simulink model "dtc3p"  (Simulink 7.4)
settings: Solver=ode45  StartTime=0.0  StopTime=.03  MaxStep=2e-5  RelTol=1e-3
undefined symbols (not defined in the file or in its folder): a

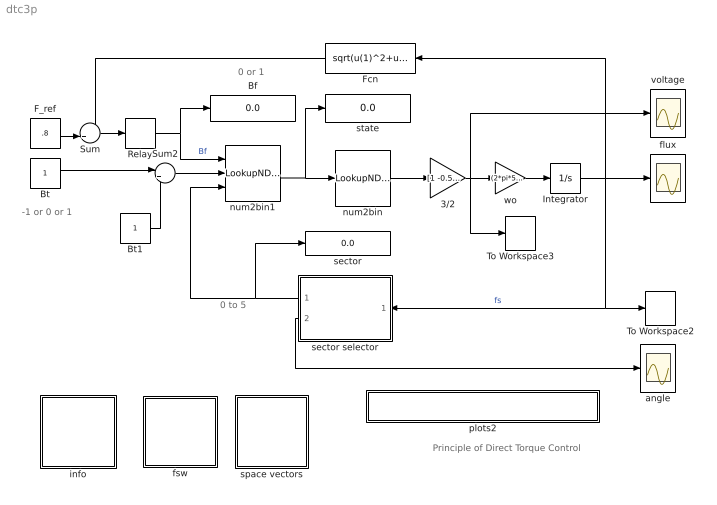
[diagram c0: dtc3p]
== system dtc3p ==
  note: Principle of Direct Torque Control
  note: -1 or 0 or 1
  note: 0 to 5
  note: 0 or 1
  3/2 : Gain  Gain=[1 -0.5 -0.5;0 sqrt(3)/2 -sqrt(3)/2]  Multiplication=Matrix(K*u)  ParameterDataType=sfix(16)  ParameterScaling=2^0  OutDataType=sfix(16)  OutScaling=2^0
  Bf : Display
  Bt : Constant  OutDataType=sfix(16)  OutScaling=2^0
  Bt1 : Constant  OutDataType=sfix(16)  OutScaling=2^0
  F_ref : Constant  Value=.8  OutDataType=sfix(16)  OutScaling=2^0
  Fcn : Fcn  Expr=sqrt(u(1)^2+u(2)^2)
  Integrator : Integrator  InitialCondition=[1 0]
  Relay : Relay  OnSwitchValue=.02  OffSwitchValue=-.02  OutDataType=sfix(16)  OutScaling=2^0
  Sum : Sum  Inputs=-+|  OutDataType=sfix(16)  OutScaling=2^0
  Sum2 : Sum  Inputs=|++  OutDataType=sfix(16)  OutScaling=2^0
  To Workspace2 : ToWorkspace  VariableName=f_ab  SampleTime=-1  SaveFormat=Array
  To Workspace3 : ToWorkspace  VariableName=f  SampleTime=-1  SaveFormat=Array
  angle : Scope
  flux : Scope
  fsw : Subsystem
  info : Subsystem
  num2bin : LookupNDDirect  InputsSelectThisObjectFromTable=Column  Table=[0 0 0;1 0 0;0 1 0;1 1 0;0 0 1;1 0 1;0 1 1;1 1 1]'  ActionForOutOfRangeInput=Error
  num2bin1 : LookupNDDirect  NumberOfTableDimensions=3  Table=a  ActionForOutOfRangeInput=Error
  plots2 : Subsystem
  sector : Display
  sector selector : Subsystem
  space vectors : Subsystem
  state : Display
  voltage : Scope
  wo : Gain  Gain=(2*pi*50)  ParameterDataType=sfix(16)  ParameterScaling=2^0  OutDataType=sfix(16)  OutScaling=2^0
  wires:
  num2bin1/1 -> state/1, num2bin/1
  num2bin/1 -> 3/2/1
  F_ref/1 -> Sum/2
  Sum/1 -> Relay/1
  Relay/1 -> Bf/1, num2bin1/1  "Bf"
  Fcn/1 -> Sum/1
  wo/1 -> Integrator/1
  3/2/1 -> wo/1, voltage/1, To Workspace3/1
  Integrator/1 -> Fcn/1, flux/1, sector selector/1(fs), To Workspace2/1  "fs"
  sector selector/1(sector) -> sector/1, num2bin1/3
  Sum2/1 -> num2bin1/2
  Bt/1 -> Sum2/1
  Bt1/1 -> Sum2/2
  sector selector/2(angle) -> angle/1

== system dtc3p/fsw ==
  note: Script files
  note: This collection of demonstrations is designed to illustrate the use of MATLAB for the simulation of the steady-state characteristics of ac machines under balanced and unbalanced conditions of operation.

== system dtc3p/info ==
  note: Principle of direct torque control of an induction motor
  note: This demo shows how to produce a rotating flux vector of specified magnitude F_ref using the principle of direct torque control: a) Bt = 1 establishes a positively rotating wave (counterclockwize) b) Bt = -1 establishes a negatively rotating wave (clockwize) c) Bt = 0 keeps the flux vector fixed in its original state Before running, double click the Switching Table block. Observe the effect of changing the magnitude of F_ref and/or wo (gain preceding the integrator) upon the speed (frequency) of the rotating space vector.

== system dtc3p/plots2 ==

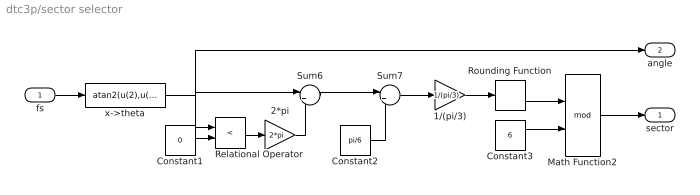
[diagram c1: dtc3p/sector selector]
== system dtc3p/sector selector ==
  fs : Inport  OutDataType=sfix(16)  OutScaling=2^0
  1/(pi/3) : Gain  Gain=1/(pi/3)  ParameterDataType=sfix(16)  ParameterScaling=2^0  OutDataType=sfix(16)  OutScaling=2^0
  2*pi : Gain  Gain=2*pi  ParameterDataType=sfix(16)  ParameterScaling=2^0  OutDataType=sfix(16)  OutScaling=2^0
  Constant1 : Constant  Value=0  OutDataType=sfix(16)  OutScaling=2^0
  Constant2 : Constant  Value=pi/6  OutDataType=sfix(16)  OutScaling=2^0
  Constant3 : Constant  Value=6  OutDataType=sfix(16)  OutScaling=2^0
  Math Function2 : Math  Operator=mod
  Relational Operator : RelationalOperator  Operator=<
  Rounding Function : Rounding
  Sum6 : Sum  Inputs=|++  OutDataType=sfix(16)  OutScaling=2^0
  Sum7 : Sum  Inputs=|++  OutDataType=sfix(16)  OutScaling=2^0
  x->theta : Fcn  Expr=atan2(u(2),u(1))
  sector : Outport
  angle : Outport  Port=2
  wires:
  Constant1/1 -> Relational Operator/2
  Relational Operator/1 -> 2*pi/1
  2*pi/1 -> Sum6/2
  Sum6/1 -> Sum7/1
  Constant2/1 -> Sum7/2
  Sum7/1 -> 1/(pi/3)/1
  1/(pi/3)/1 -> Rounding Function/1
  Rounding Function/1 -> Math Function2/1
  Constant3/1 -> Math Function2/2
  fs/1 -> x->theta/1
  Math Function2/1 -> sector/1
  x->theta/1 -> Relational Operator/1, Sum6/1, angle/1

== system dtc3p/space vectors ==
